TYPE series5x_PDout :
STRUCT
	TextToDisplay : STRING(5); //value you write to
	stringToBytes : StringToBytes; // link raw data
	DisplayedNumber : UDINT; //value you write to
	displayedNumberStuct : DisplayedNumber_Struct; //link raw data 
	TextColor AT %Q* : USINT; 
	TextSelect AT %Q*: USINT;
	ActiveScenes : INT; // value you write to
	activeScenesSctruct : ActiveScenes_Struct; //link raw data 
	Mode AT %Q*: USINT;
END_STRUCT
END_TYPE
